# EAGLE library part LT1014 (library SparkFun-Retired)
Precision quad op-amp. I/O range includes negative rail. Dead Prototype: IC-08606 TODO: fix symbol
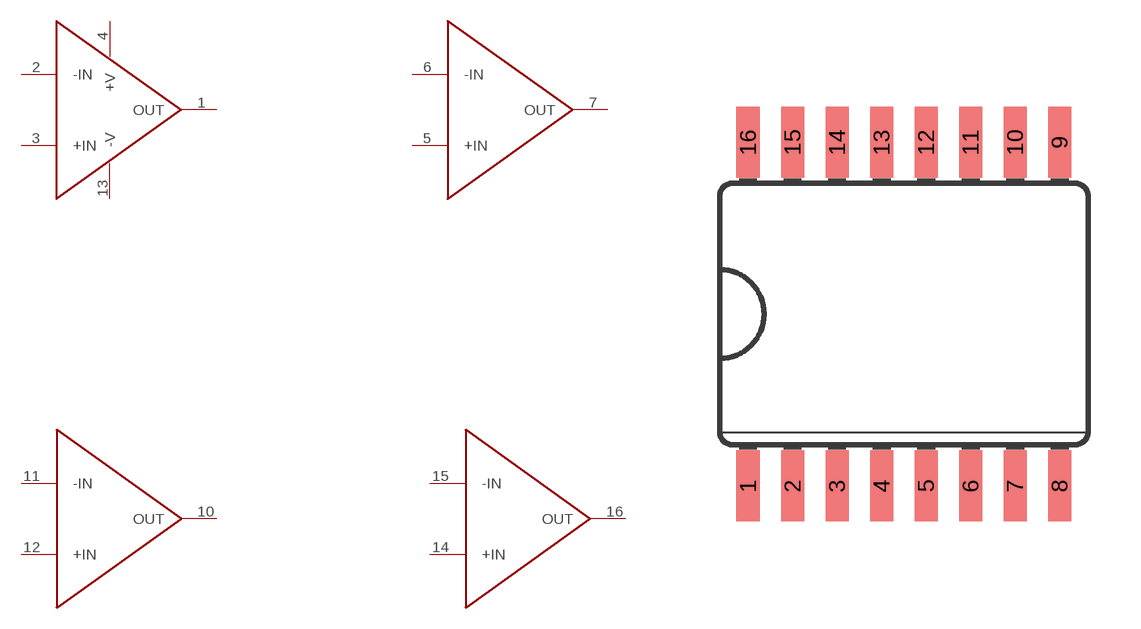
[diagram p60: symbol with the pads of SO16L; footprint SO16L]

Designator prefix -; gates G1=LT1014 G2=LT1014_2 G3=LT1014_2 G4=LT1014_2

## LT1014  [SO16L]
1  G1:OUT  out
2  G1:-IN  in
3  G1:+IN  in
4  G1:+V  pwr
5  G2:+IN  pwr
6  G2:-IN  pwr
7  G2:OUT  pwr
10  G3:OUT  pwr
11  G3:-IN  pwr
12  G3:+IN  pwr
13  G1:-V  pwr
14  G4:+IN  pwr
15  G4:-IN  pwr
16  G4:OUT  pwr

## Footprint SO16L (pad centres in mm)
Small Outline Package .300 SIOC Source: http://www.maxim-ic.com/cgi-bin/packages?pkg=16%2FSOIC%2E300&Type=Max
smd 0.66 x 2.032: 1 -4.445,-4.902; 2 -3.175,-4.902; 3 -1.905,-4.902; 4 -0.635,-4.902; 5 0.635,-4.902; 6 1.905,-4.902; 7 3.175,-4.902; 8 4.445,-4.902; 9 4.445,4.902; 10 3.175,4.902; 11 1.905,4.902; 12 0.635,4.902; 13 -0.635,4.902; 14 -1.905,4.902; 15 -3.175,4.902; 16 -4.445,4.902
